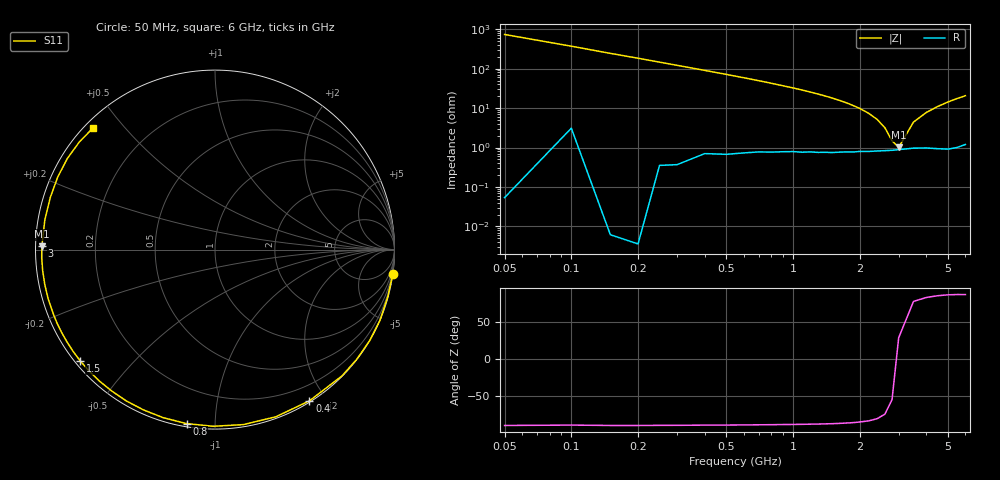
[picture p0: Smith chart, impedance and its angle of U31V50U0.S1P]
! SIEMENS Discrete & RF Semiconductors
! BBY53-02W
! Si Tuning Diode in SCD-80
! VR = 1.5 V
! S-Parameters:  September  1997
# GHz  S  MA  R  50
!  f  S11
! GHz  MAG  ANG
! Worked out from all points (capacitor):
!   34 points, 50 MHz to 6 GHz, reference 50 ohm
!   read as one part to ground: C = 4.34 pF near 50 MHz
!   lowest |Z| = 1.01 ohm at 3 GHz (marker M1)
!   series resonance near 2.944 GHz, so ESL is about 670 pH
!   S11 on the Smith chart (normalised r, x): 50 MHz: 0, -15; 400 MHz: 0.01, -1.80; 800 MHz: 0.02, -0.85; 1.5 GHz: 0.01, -0.36; 3 GHz: 0.02, +0.01; 6 GHz: 0.02, +0.41
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0.05  1 -7.8
0.1  0.9978 -15.4
0.15  1 -23.2
0.2  1 -30.5
0.25  0.9985 -37.8
0.3  0.9979 -44.8
0.4  0.9934 -58.0
0.5  0.9912 -70.0
0.6  0.9878 -80.8
0.7  0.9845 -90.6
0.8  0.9823 -99.3
0.9  0.9799 -107.2
1  0.978 -114.0
1.1  0.9773 -120.3
1.2  0.9756 -126.1
1.3  0.9753 -131.3
1.5  0.9739 -140.4
1.6  0.9728 -144.4
1.9  0.9708 -154.9
2.2  0.9693 -163.4
2.4  0.9681 -168.4
3  0.9651 178.9
3.5  0.9624 170.1
4  0.9625 162.5
4.5  0.9649 155.3
5  0.9668 148.3
5.5  0.9648 141.6
6  0.9598 135.3
